FUNCTION "PartContr.Loader" : VOID
TITLE =Part Control
VERSION : 0.1

BEGIN
NETWORK
TITLE =PRESENZA FOGLIO SU VENTOSE SFOGLIATORE
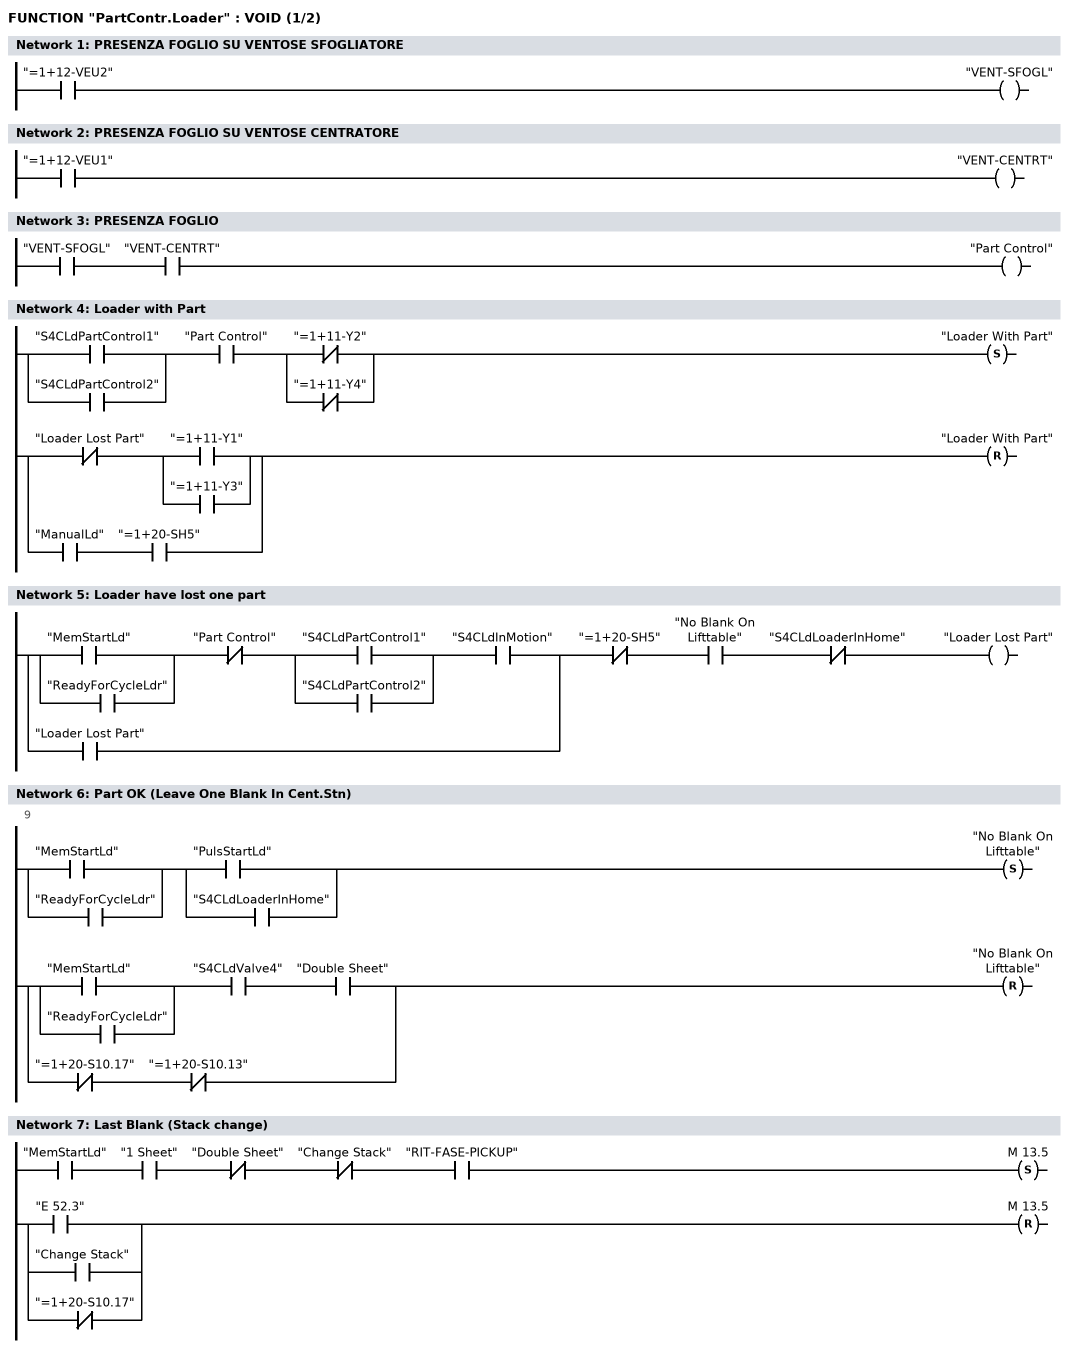
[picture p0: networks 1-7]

      U     "=1+12-VEU2";
      =     "VENT-SFOGL";
NETWORK
TITLE =PRESENZA FOGLIO SU VENTOSE CENTRATORE

      U     "=1+12-VEU1";
      =     "VENT-CENTRT";
NETWORK
TITLE =PRESENZA FOGLIO

      U     "VENT-SFOGL";
      U     "VENT-CENTRT";
      =     "Part Control";
NETWORK
TITLE =Loader with Part

      U(    ;
      O     "S4CLdPartControl1";
      O     "S4CLdPartControl2";
      )     ;
      U     "Part Control";
      U(    ;
      ON    "=1+11-Y2";
      ON    "=1+11-Y4";
      )     ;
      S     "Loader With Part";
      U(    ;
      UN    "Loader Lost Part";
      U(    ;
      O     "=1+11-Y1";
      O     "=1+11-Y3";
      )     ;
      O     ;
      U     "ManualLd";
      U     "=1+20-SH5";
      )     ;
      R     "Loader With Part";
      NOP   0;
NETWORK
TITLE =Loader have lost one part

      U(    ;
      U(    ;
      O     "MemStartLd";
      O     "ReadyForCycleLdr";
      )     ;
      UN    "Part Control";
      U(    ;
      O     "S4CLdPartControl1";
      O     "S4CLdPartControl2";
      )     ;
      U     "S4CLdInMotion";
      O     "Loader Lost Part";
      )     ;
      UN    "=1+20-SH5";
      U     "No Blank On Lifttable";
      UN    "S4CLdLoaderInHome";
      =     "Loader Lost Part";
NETWORK
TITLE =Part OK (Leave One Blank In Cent.Stn)
//9
      U(    ;
      O     "MemStartLd";
      O     "ReadyForCycleLdr";
      )     ;
      U(    ;
      O     "PulsStartLd";
      O     "S4CLdLoaderInHome";
      )     ;
      S     "No Blank On Lifttable";
      U(    ;
      U(    ;
      O     "MemStartLd";
      O     "ReadyForCycleLdr";
      )     ;
      U     "S4CLdValve4";
      U     "Double Sheet";
      O     ;
      UN    "=1+20-S10.17";
      UN    "=1+20-S10.13";
      )     ;
      R     "No Blank On Lifttable";
      NOP   0;
NETWORK
TITLE =Last Blank (Stack change)

      U     "MemStartLd";
      U     "1 Sheet";
      UN    "Double Sheet";
      UN    "Change Stack";
      U     "RIT-FASE-PICKUP";
      S     M     13.5;
      U(    ;
      O     "E 52.3";
      O     "Change Stack";
      ON    "=1+20-S10.17";
      )     ;
      R     M     13.5;
      NOP   0;
NETWORK
TITLE =Check If Not Last Blank
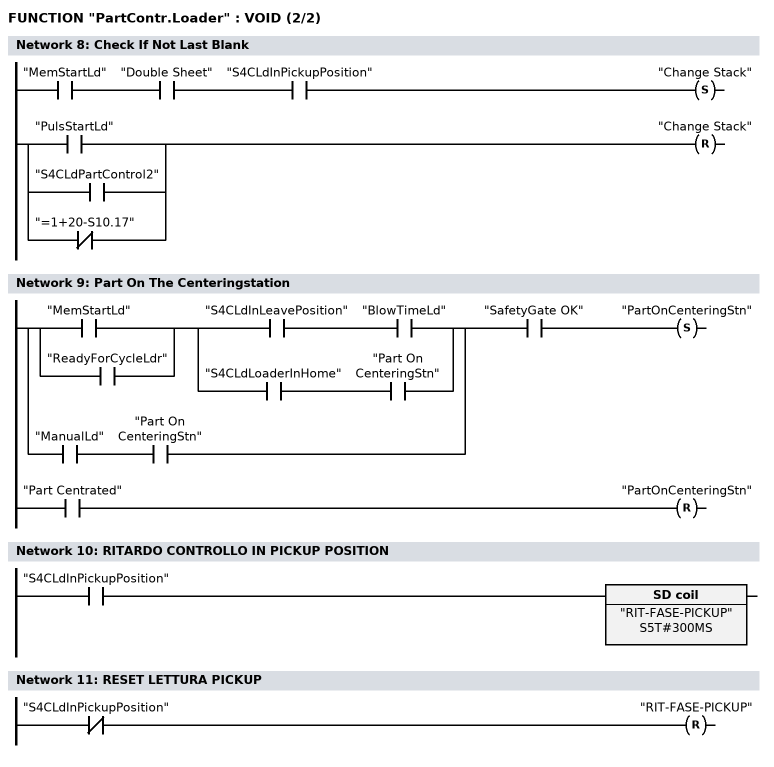
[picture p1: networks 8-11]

      U     "MemStartLd";
      U     "Double Sheet";
      U     "S4CLdInPickupPosition";
      S     "Change Stack";
      U(    ;
      O     "PulsStartLd";
      O     "S4CLdPartControl2";
      ON    "=1+20-S10.17";
      )     ;
      R     "Change Stack";
      NOP   0;
NETWORK
TITLE =Part On The Centeringstation

      U(    ;
      U(    ;
      O     "MemStartLd";
      O     "ReadyForCycleLdr";
      )     ;
      U(    ;
      U     "S4CLdInLeavePosition";
      U     "BlowTimeLd";
      O     ;
      U     "S4CLdLoaderInHome";
      U     "Part On CenteringStn";
      )     ;
      O     ;
      U     "ManualLd";
      U     "Part On CenteringStn";
      )     ;
      U     "SafetyGate OK";
      S     "PartOnCenteringStn";
      U     "Part Centrated";
      R     "PartOnCenteringStn";
      NOP   0;
NETWORK
TITLE =RITARDO CONTROLLO IN PICKUP POSITION

      U     "S4CLdInPickupPosition";
      L     S5T#300MS;
      SE    "RIT-FASE-PICKUP";
NETWORK
TITLE =RESET LETTURA PICKUP

      UN    "S4CLdInPickupPosition";
      R     "RIT-FASE-PICKUP";


END_FUNCTION

